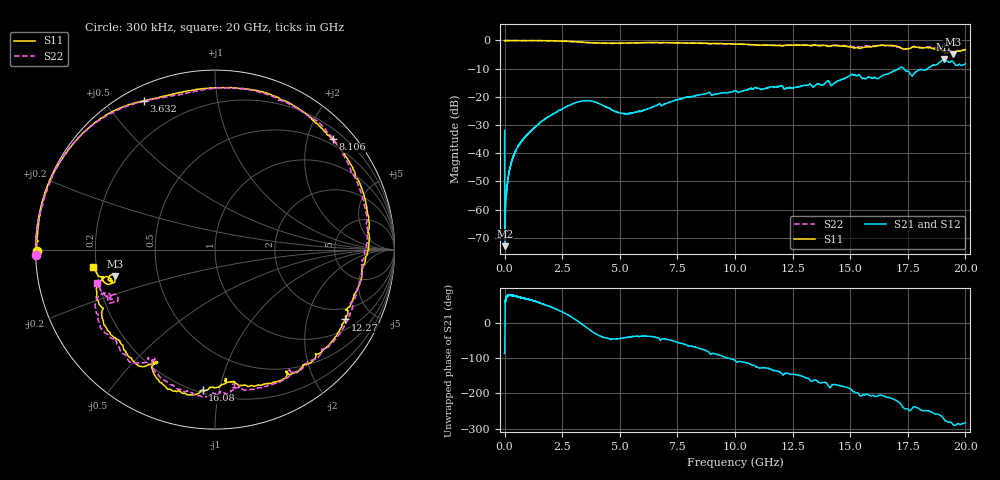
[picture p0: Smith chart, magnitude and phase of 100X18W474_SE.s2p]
!{100X18W474_SE}
!Johanson Technology Inc.
!www.johansontechnology.com
!Test Board Conditions:
!Substrate Type  RO4350B
!Substrate Thickness  21 mil
!Substrate Dk  3.66
!TL Type: GCPW
!TL Trace Width  40 mil
!TL Gap  20 mil
!PART MODE SINGLE ENDED (AKA BYPASS)
!DUT TOPOLOGY	SERIES-SHUNT
!Mounting Pad LxW  120x40 mil
! Created Wed Oct 27 11:12:16 2021
# hz S ma R 50
! 2 Port Network Data from SP1.SP block
! freq  magS11  angS11  magS21  angS21  magS12  angS12  magS22  angS22
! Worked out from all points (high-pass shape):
!   20001 points, 300 kHz to 20 GHz, reference 50 ohm
!   highest |S21| = -6.69 dB at 19.07 GHz (marker M1); lowest = -73.0 dB at 13.3 MHz (marker M2)
!   |S21| within 3 dB of the highest: 17.16 GHz to 17.29 GHz (125.4 MHz wide, 0.728 % of centre); 18.41 GHz to end of sweep
!   lowest |S11| = -4.8 dB at 19.45 GHz (marker M3), VSWR 3.73, Z = 13.6 - j6.03 ohm
!   |S11| at or under -10 dB: nowhere
!   |S22| runs from -4.4 to 0.0 dB; largest |S21 - S12| = 0.013
!   S11 on the Smith chart (normalised r, x): 300 kHz: 0.00, -0.00; 3.632 GHz: 0.06, +0.63; 8.106 GHz: 0.39, +2.48; 12.27 GHz: 1.42, -3.44; 16.08 GHz: 0.22, -0.89; 20 GHz: 0.19, -0.07
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300000  0.9919 -179.6  0.0255 -87.7  0.02567 -88.9  0.9997 -178.2
1.33e7  0.994 179.7  0.0002246 -37.9  0.00024 -34.9  1 179.8
1.023e8  0.9928 178.3  0.00258 74.9  0.00255 76.5  1 178.2
1.873e8  0.9912 176.8  0.004519 76.4  0.004443 77.6  0.9999 176.8
3.323e8  0.9929 174.2  0.007884 77.0  0.007739 76.2  0.9991 174.1
8.093e8  0.9972 166.1  0.01772 68.7  0.01796 68.8  0.9936 165.7
1.7553e9  0.9897 148.4  0.04047 50.1  0.04047 50.3  0.9914 148.4
3.3343e9  0.9346 119.9  0.08416 -3.8  0.08434 -3.8  0.9277 118.8
3.6323e9  0.9182 115.6  0.08561 -18.1  0.08579 -18.1  0.9122 114.0
5.1993e9  0.9004 91.9  0.05043 -43.1  0.05066 -43.1  0.8934 93.8
6.6673e9  0.9167 67.3  0.0731 -42.9  0.07311 -43.3  0.9127 68.0
8.1063e9  0.8983 43.2  0.1001 -66.7  0.09936 -66.6  0.9032 43.8
1.00003e10  0.8611 7.3  0.1284 -107.9  0.1291 -107.7  0.8566 10.0
1.22723e10  0.8239 -28.2  0.1429 -144.0  0.1406 -143.6  0.834 -24.8
1.33343e10  0.8122 -46.1  0.1569 -166.5  0.1576 -166.0  0.815 -43.2
1.51013e10  0.7473 -81.5  0.2495 166.2  0.2486 165.6  0.7791 -80.3
1.60773e10  0.7862 -95.0  0.2204 151.0  0.221 151.0  0.801 -90.6
1.66673e10  0.819 -105.4  0.2579 147.9  0.2555 150.1  0.8057 -103.2
1.84323e10  0.7467 -145.8  0.3331 109.7  0.3355 109.4  0.771 -146.1
1.90743e10  0.6239 -166.0  0.4632 86.2  0.4614 86.3  0.6539 -158.3
1.94523e10  0.577 -165.2  0.4247 71.7  0.4198 71.7  0.6066 -155.2
2e10  0.6804 -172.3  0.3877 76.2  0.3872 75.3  0.6834 -164.4
